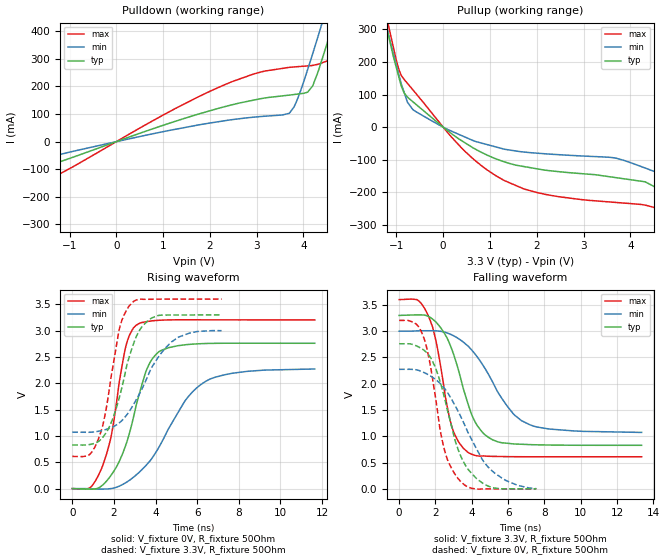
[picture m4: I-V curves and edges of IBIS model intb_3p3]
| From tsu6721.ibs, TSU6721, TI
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|   intb_3p3 Model
[Model]   intb_3p3
Model_type   Output
Polarity   Non-Inverting
Vmeas = 1.65
Vref = 1.65
Cref = 2pF
Rref = 50
|   typ   min   max
C_comp   2.588e-12   2.461e-12   2.799e-12
[Voltage Range]   3.3   3   3.6
|Ambient Temperature   25   85   -40
|Junction Temperature
[Temperature Range]   27   125   -40
[Pullup Reference]   3.3   3   3.6
[Pulldown Reference]   0   0   0
[Power Clamp Reference]   3.3   3   3.6
[GND Clamp Reference]   0   0   0
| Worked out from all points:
|   slope of the pulldown table from 0 to 0.495 V, typ, clamps not added: 16.6 ohm
|   slope of the pullup table from 0 to 0.495 V, typ, clamps not added: 9.78 ohm
|   falling waveform, V_fixture 3.3V, R_fixture 50Ohm: 20-80 % time 1.39ns typ, 2.15ns min, 985ps max; typ from 3.3 V to 0.829 V
|   rising waveform, V_fixture 0V, R_fixture 50Ohm: 20-80 % time 1.23ns typ, 2.16ns min, 866ps max; typ from 0 V to 2.76 V
|   rising waveform, V_fixture 3.3V, R_fixture 50Ohm: 20-80 % time 1.06ns typ, 1.64ns min, 774ps max; typ from 0.829 V to 3.3 V
|   falling waveform, V_fixture 0V, R_fixture 50Ohm: 20-80 % time 1.39ns typ, 2.11ns min, 984ps max; typ from 2.76 V to 0.001 V
[Pulldown]
|   Voltage   I(typ)   I(min)   I(max)
-3.3V     -197.4mA   -130mA     -309.5mA
1.782V    101.2mA    61.31mA    164.7mA
2.934V    150.4mA    88.7mA     245mA
3.69V     168.4mA    102.3mA    268.9mA
3.855V    171.9mA    147mA      271.3mA
4.089V    179.2mA    261mA      274.3mA
4.198V    202.1mA    318.9mA    276.2mA
4.316V    255.2mA    384.1mA    280.4mA
4.468V    336mA      469.4mA    289.9mA
4.572V    395.1mA    528.4mA    313.6mA
4.824V    540.8mA    673.9mA    447.6mA
6.6V      1.633A     1.734A     1.567A
[Pullup]
|   Voltage   I(typ)   I(min)   I(max)
-3.3V     1.653A     1.594A     1.765A
-1.217V   311mA      313.2mA    342.1mA
-1.125V   254.1mA    258.9mA    283.6mA
-894.3mV  125.5mA    132.3mA    158.4mA
-648mV    77.92mA    53.78mA    114.6mA
478.8mV   -49.17mA   -31.17mA   -75.98mA
1.318V    -106.9mA   -68mA      -164.6mA
3.702V    -155.2mA   -95.49mA   -231.2mA
4.316V    -167.7mA   -125.4mA   -239.2mA
4.892V    -214.4mA   -156.9mA   -284.1mA
6V        -306.6mA   -217.8mA   -427.4mA
6.6V      -356.6mA   -250.8mA   -505mA
[Ramp]
R_load = 50
|   typ   min   max
dV/dt_r   1.65636/1.22589e-09   1.36482/2.15903e-09   1.92298/8.6499e-10
dV/dt_f   1.48248/1.38567e-09   1.15775/2.1447e-09   1.79319/9.80308e-10
[Falling Waveform]
V_fixture = 3.3V
V_fixture_min = 3V
V_fixture_max = 3.6V
R_fixture = 50Ohm
|   Time   V(typ)   V(min)   V(max)
0s        3.3V       3V         3.6V
975ps     3.31V      3.006V     3.601V
1.575ns   3.287V     3.009V     3.314V
2.025ns   3.173V     3.006V     2.817V
2.9ns     2.655V     2.93V      1.186V
3.825ns   1.582V     2.705V     688mV
4.775ns   1.016V     2.264V     623.9mV
5.925ns   869.6mV    1.586V     614mV
6.725ns   849.7mV    1.3V       611.8mV
13.35ns   829.2mV    1.074V     611.4mV
[Rising Waveform]
V_fixture = 0V
V_fixture_min = 0V
V_fixture_max = 0V
R_fixture = 50Ohm
|   Time   V(typ)   V(min)   V(max)
0s        5.863nV    303.6nV    247pV
825ps     -10.26mV   -3.865mV   7.461mV
1.45ns    64.68mV    -8.639mV   424.2mV
1.875ns   259.3mV    978.3uV    1.011V
2.55ns    803.5mV    107.3mV    2.664V
3.05ns    1.546V     252mV      3.097V
3.525ns   2.21V      433mV      3.168V
4.075ns   2.57V      726.8mV    3.195V
6.4ns     2.756V     2.035V     3.206V
11.65ns   2.761V     2.272V     3.205V
[Rising Waveform]
V_fixture = 3.3V
V_fixture_min = 3V
V_fixture_max = 3.6V
R_fixture = 50Ohm
|   Time   V(typ)   V(min)   V(max)
0s        829.2mV    1.07V      611.4mV
800ps     835.1mV    1.07V      637.9mV
1.25ns    893.5mV    1.089V     937.9mV
1.6ns     1.047V     1.121V     1.454V
2.25ns    1.715V     1.247V     3.014V
2.85ns    2.644V     1.536V     3.52V
3.2ns     2.986V     1.779V     3.596V
3.625ns   3.184V     2.133V     3.596V
4.775ns   3.297V     2.788V     3.6V
7.175ns   3.3V       3V         3.6V
[Falling Waveform]
V_fixture = 0V
V_fixture_min = 0V
V_fixture_max = 0V
R_fixture = 50Ohm
|   Time   V(typ)   V(min)   V(max)
0s        2.761V     2.275V     3.205V
925ps     2.725V     2.267V     3.14V
1.325ns   2.648V     2.221V     2.904V
1.7ns     2.512V     2.153V     2.381V
2.45ns    1.797V     1.933V     803mV
2.75ns    1.374V     1.785V     482.4mV
3.275ns   722.9mV    1.457V     185.1mV
3.8ns     369.9mV    1.067V     34.28mV
4.975ns   43.35mV    387.3mV    418.7uV
7.55ns    877.1uV    4.667mV    -40.23uV
